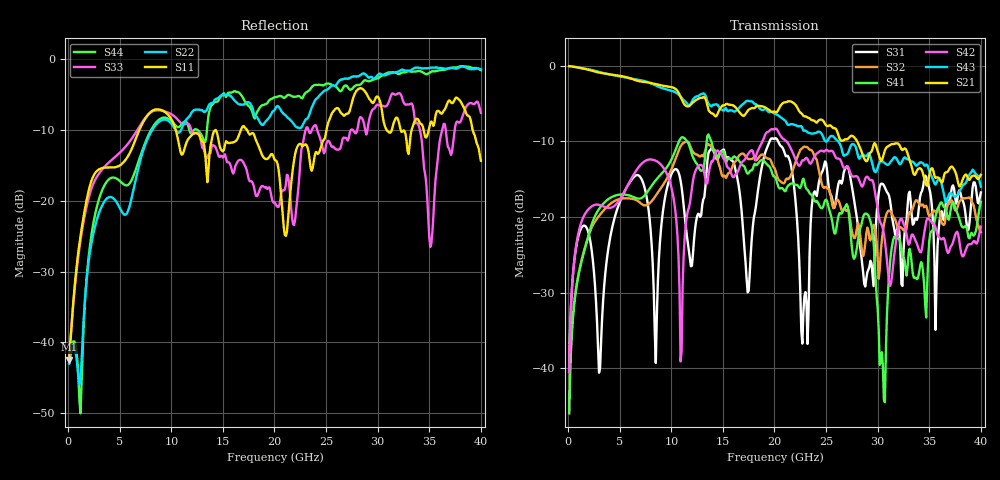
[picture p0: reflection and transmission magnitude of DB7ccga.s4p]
! ADC12DJ3200QML-SP
! 196-pin NWE package
! CCGA Ceramic Package with columns (ceramic column grid array)
! Texas Instruments 4/21/2021
! Single-ended  S-parameters
! PORT#  PORT_NAME  NET_NAME
! PORT1:  DAxN.DIEBUMP DAxN
! PORT2:  DAxN.BGA  DAxN
! PORT3:  DAxP.DIEBUMP DAxP
! PORT4:  DAxP.BGA  DAxP
! Touchstone Ver. 1.0
! Number of ports is 4
# Hz	S	MA	R	50.000000
! SCATTERING PARAMETERS  :
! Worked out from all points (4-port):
!   400 points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, 100 MHz to 40 GHz, reference 50 ohm
!   strongest paths, dB at 100 MHz, 10.1 GHz, 20.1 GHz, 30.1 GHz, 40 GHz:
!     S21: -0.1, -2.9, -6.2, -11.8, -14.4
!     S43: -0.1, -3.3, -6.4, -13.0, -16.0
!     S42: -40.5, -16.6, -8.3, -19.9, -21.3
!     S41: -46.0, -12.2, -14.8, -34.9, -18.0
!     S32: -46.0, -13.4, -13.9, -28.2, -22.0
!     S31: -40.5, -14.1, -9.6, -16.8, -16.8
!   lowest |S11| = -42.5 dB at 100 MHz (marker M1), VSWR 1.02, Z = 50.7 + j0.148 ohm
!   |S11| at or under -10 dB: start of sweep to 6.895 GHz; 10.43 GHz to 14.27 GHz (3.842 GHz wide, 31.1 % of centre); 17.34 GHz to 25.04 GHz (7.699 GHz wide, 36.3 % of centre)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
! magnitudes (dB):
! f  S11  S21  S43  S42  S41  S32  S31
! 100 MHz  -42.5  -0.1  -0.1  -40.5  -46.0  -46.0  -40.5
! 8.3 GHz  -7.2  -2.4  -2.5  -12.5  -15.5  -17.6  -29.7
! 10.9 GHz  -13.1  -4.1  -4.1  -39.1  -9.6  -10.7  -15.2
! 14.4 GHz  -10.2  -6.6  -5.1  -11.3  -12.1  -11.9  -12.4
! 22.7 GHz  -12.3  -6.4  -8.2  -12.5  -15.2  -10.9  -36.8
! 30.7 GHz  -9.4  -11.2  -12.9  -23.2  -44.5  -20.4  -16.1
! 40 GHz  -14.3  -14.4  -16.0  -21.3  -18.0  -22.0  -16.8
